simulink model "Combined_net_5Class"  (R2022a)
settings: Solver=FixedStepAuto  StartTime=0.0  StopTime=simtime  FixedStep=1  RelTol=1e-3
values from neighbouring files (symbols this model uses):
  simtime = length(SOC_CC{1, 1})    [Data_preparation.m]    (also in SimulationCycle.m = cell2mat(simtime_og(i)))
  SOH_predict = double(ans.SOHout(simtime))    [SimulationCycle.m]
undefined symbols (not defined in the file or in its folder): dSOC_mu_CC, dSOC_sig_CC, dv_mu_CC, dv_sig_CC, SOC_mu_CC, SOC_sig_CC, SOE_mu_CC, SOE_sig_CC
libraries: neural x183, deeplib x1
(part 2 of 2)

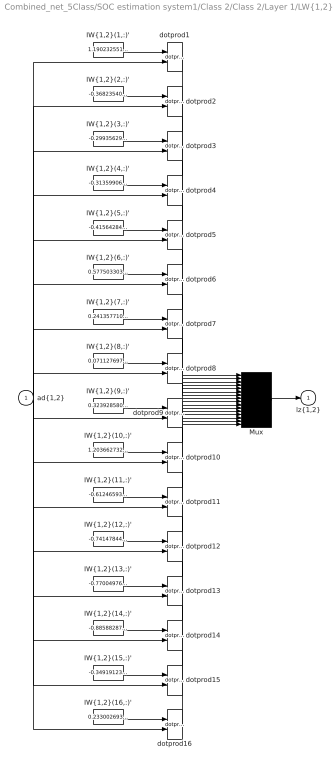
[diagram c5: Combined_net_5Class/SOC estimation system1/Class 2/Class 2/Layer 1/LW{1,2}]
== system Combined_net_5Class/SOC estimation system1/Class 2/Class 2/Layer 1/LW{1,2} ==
  "ad{1,2}" : Inport  PortDimensions=1  SampleTime=1
  "IW{1,2}(1,:)'" : Constant  Value=1.1902325515607079520208344547427259385585784912109375
  "IW{1,2}(10,:)'" : Constant  Value=1.2036627323236273046092037475318647921085357666015625
  "IW{1,2}(11,:)'" : Constant  Value=-0.61246593854063480222293947008438408374786376953125
  "IW{1,2}(12,:)'" : Constant  Value=-0.7414784419285955774370222570723854005336761474609375
  "IW{1,2}(13,:)'" : Constant  Value=-0.7700497660412211065050769320805557072162628173828125
  "IW{1,2}(14,:)'" : Constant  Value=-0.88588287817542854529762053061858750879764556884765625
  "IW{1,2}(15,:)'" : Constant  Value=-0.34919123068833413103817520095617510378360748291015625
  "IW{1,2}(16,:)'" : Constant  Value=0.23300269357094716138334433708223514258861541748046875
  "IW{1,2}(2,:)'" : Constant  Value=-0.368235400748596009012914009872474707663059234619140625
  "IW{1,2}(3,:)'" : Constant  Value=-0.299356293819304786207879942594445310533046722412109375
  "IW{1,2}(4,:)'" : Constant  Value=-0.313599061992354710692865182863897643983364105224609375
  "IW{1,2}(5,:)'" : Constant  Value=-0.415642846228695794774665728255058638751506805419921875
  "IW{1,2}(6,:)'" : Constant  Value=0.577503303425816572058693054714240133762359619140625
  "IW{1,2}(7,:)'" : Constant  Value=0.241357710985629025923770996087114326655864715576171875
  "IW{1,2}(8,:)'" : Constant  Value=0.07112769749609226810349582592607475817203521728515625
  "IW{1,2}(9,:)'" : Constant  Value=0.32392858033215443658292542750132270157337188720703125
  Mux : Mux  Inputs=16
  dotprod{1..16} (16 alike) : neural/Weight Functions/dotprod
  "lz{1,2}" : Outport
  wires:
  "IW{1,2}(1,:)'"/1 -> dotprod1/1
  "ad{1,2}"/1 -> dotprod1/2, dotprod2/2, dotprod3/2, dotprod4/2, dotprod5/2, dotprod6/2, dotprod7/2, dotprod8/2, dotprod9/2, dotprod10/2, dotprod11/2, dotprod12/2, dotprod13/2, dotprod14/2, dotprod15/2, dotprod16/2
  dotprod1/1 -> Mux/1
  "IW{1,2}(2,:)'"/1 -> dotprod2/1
  dotprod2/1 -> Mux/2
  "IW{1,2}(3,:)'"/1 -> dotprod3/1
  dotprod3/1 -> Mux/3
  "IW{1,2}(4,:)'"/1 -> dotprod4/1
  dotprod4/1 -> Mux/4
  "IW{1,2}(5,:)'"/1 -> dotprod5/1
  dotprod5/1 -> Mux/5
  "IW{1,2}(6,:)'"/1 -> dotprod6/1
  dotprod6/1 -> Mux/6
  "IW{1,2}(7,:)'"/1 -> dotprod7/1
  dotprod7/1 -> Mux/7
  "IW{1,2}(8,:)'"/1 -> dotprod8/1
  dotprod8/1 -> Mux/8
  "IW{1,2}(9,:)'"/1 -> dotprod9/1
  dotprod9/1 -> Mux/9
  "IW{1,2}(10,:)'"/1 -> dotprod10/1
  dotprod10/1 -> Mux/10
  "IW{1,2}(11,:)'"/1 -> dotprod11/1
  dotprod11/1 -> Mux/11
  "IW{1,2}(12,:)'"/1 -> dotprod12/1
  dotprod12/1 -> Mux/12
  "IW{1,2}(13,:)'"/1 -> dotprod13/1
  dotprod13/1 -> Mux/13
  "IW{1,2}(14,:)'"/1 -> dotprod14/1
  dotprod14/1 -> Mux/14
  "IW{1,2}(15,:)'"/1 -> dotprod15/1
  dotprod15/1 -> Mux/15
  "IW{1,2}(16,:)'"/1 -> dotprod16/1
  dotprod16/1 -> Mux/16
  Mux/1 -> "lz{1,2}"/1

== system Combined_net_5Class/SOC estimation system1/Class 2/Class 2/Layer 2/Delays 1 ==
  "p{2}" : Inport  PortDimensions=16  SampleTime=1
  mux : Mux  Inputs=1
  "pd{2,1}" : Outport
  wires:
  "p{2}"/1 -> mux/1
  mux/1 -> "pd{2,1}"/1

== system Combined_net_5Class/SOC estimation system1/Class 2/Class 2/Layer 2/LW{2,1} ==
  "ad{2,1}" : Inport  PortDimensions=16  SampleTime=1
  "IW{2,1}(1,:)'" : Constant  Value=[0.0007484560447357057992590068096205868641845881938934326171875;0.428302012501528384103011148908990435302257537841796875;-0.76136838015648000688173624439514242112636566162109375;-2.041090507574473189578156961943022906780242919921875;-1.5560079275295770617759671949897892773151397705078125;0.0002346400169689350358008528285580496230977587401866912841796875;0.00025834410646503381571437163444215912022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
  Mux : Mux  Inputs=1
  dotprod1 : neural/Weight Functions/dotprod
  "lz{2,1}" : Outport
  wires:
  "IW{2,1}(1,:)'"/1 -> dotprod1/1
  "ad{2,1}"/1 -> dotprod1/2
  dotprod1/1 -> Mux/1
  Mux/1 -> "lz{2,1}"/1

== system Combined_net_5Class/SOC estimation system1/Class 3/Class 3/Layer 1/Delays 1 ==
  "p{1}" : Inport  PortDimensions=3  SampleTime=1
  Delay 1 : UnitDelay  InitialCondition=pi_input_1_delayed_1
  mux : Mux  Inputs=2
  "pd{1,1}" : Outport
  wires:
  "p{1}"/1 -> Delay 1/1, mux/1
  Delay 1/1 -> mux/2
  mux/1 -> "pd{1,1}"/1

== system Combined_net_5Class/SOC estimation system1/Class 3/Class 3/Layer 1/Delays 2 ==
  "p{1}" : Inport  PortDimensions=1  SampleTime=1
  Delay 1 : UnitDelay  InitialCondition=ai_layer_2_delayed_1
  mux : Mux  Inputs=1
  "pd{1,2}" : Outport
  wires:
  "p{1}"/1 -> Delay 1/1
  Delay 1/1 -> mux/1
  mux/1 -> "pd{1,2}"/1

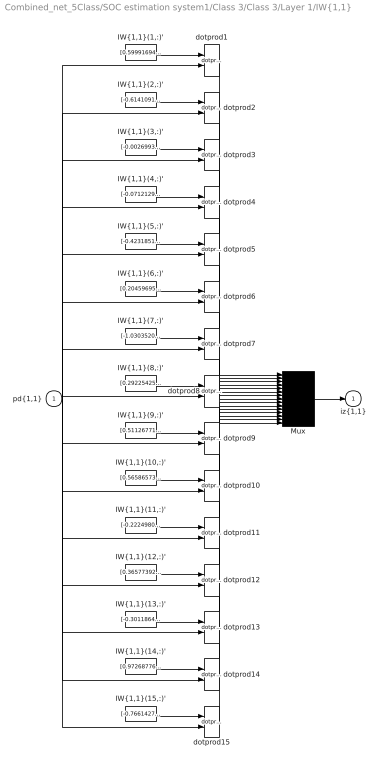
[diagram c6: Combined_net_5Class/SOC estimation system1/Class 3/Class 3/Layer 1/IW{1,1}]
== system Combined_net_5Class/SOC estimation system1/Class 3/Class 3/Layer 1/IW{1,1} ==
  "pd{1,1}" : Inport  PortDimensions=6  SampleTime=1
  "IW{1,1}(1,:)'" : Constant  Value=[0.5999169479734038912255300601827912032604217529296875;-0.380076540669565254848549784583155997097492218017578125;0.1751451252388635249079840150443487800657749176025390625;-0.581318210429382364878847511135973036289215087890625;0.388106402398013028420820091923815198242664337158203125;-0.1582639112277905157899482446737238205969333648681640625]
  "IW{1,1}(10,:)'" : Constant  Value=[0.565865737161032722468689826200716197490692138671875;-0.317511551991979945608335356155293993651866912841796875;0.71942713152451265301579041988588869571685791015625;-0.462730804023235353650278511850046925246715545654296875;-1.202674793055964475030350513407029211521148681640625;0.55537602898127691464225108575192280113697052001953125]
  "IW{1,1}(11,:)'" : Constant  Value=[-0.2224980177718796081620666882372461259365081787109375;0.0702328914913664392738468222887604497373104095458984375;-0.009460074424130826553636097742128185927867889404296875;0.2142790977150988707133905109003535471856594085693359375;-0.061660356138726273023120683092201943509280681610107421875;0.005611494475834051705309679647371012833900749683380126953125]
  "IW{1,1}(12,:)'" : Constant  Value=[0.3657739251182789974592424186994321644306182861328125;0.6914461290283744343554417355335317552089691162109375;0.004068878438489471026373589523927876143716275691986083984375;1.3485106085726688007753182318992912769317626953125;0.4634379678365778687521014944650232791900634765625;0.192226683034764700419572136524948291480541229248046875]
  "IW{1,1}(13,:)'" : Constant  Value=[-0.30118640813755892526870638903346844017505645751953125;0.460425695381792510207930035903700627386569976806640625;-0.07588917036400129323414631699051824398338794708251953125;1.275592741974297172902197416988201439380645751953125;-1.2831335957325811225615552757517434656620025634765625;-0.545358098592789719560869343695230782032012939453125]
  "IW{1,1}(14,:)'" : Constant  Value=[0.9726877674494531778037753610988147556781768798828125;0.95316906018628599905895271149347536265850067138671875;0.99977235084705673440197415402508340775966644287109375;1.0189879011847209344665543540031649172306060791015625;0.029875236411911858247503204211170668713748455047607421875;0.92824531588499337164677172040683217346668243408203125]
  "IW{1,1}(15,:)'" : Constant  Value=[-0.76614277146857745481867141279508359730243682861328125;0.790341085531665488161934263189323246479034423828125;1.167526088673049411426063670660369098186492919921875;0.52622667941697354176966427985462360084056854248046875;0.191965763204919703799333774441038258373737335205078125;-1.0897105784346734491663255539606325328350067138671875]
  "IW{1,1}(2,:)'" : Constant  Value=[-0.6141091996774454830898548607365228235721588134765625;-0.45684984466938971525706847387482412159442901611328125;0.9331109724455022291778050202992744743824005126953125;1.111277027417169716017042446765117347240447998046875;-0.27067200476342556658693183635477907955646514892578125;0.67860280468012346144490720689645968377590179443359375]
  "IW{1,1}(3,:)'" : Constant  Value=[-0.0026993480304873898080464389437338468269445002079010009765625;1.0531506048579901690942506320425309240818023681640625;-0.46427410659924195357461940147913992404937744140625;-0.06861728492135464596568539263898856006562709808349609375;-0.91250527596271047148235311397002078592777252197265625;0.44753207665025163120020579299307428300380706787109375]
  "IW{1,1}(4,:)'" : Constant  Value=[-0.0712129538313734100629659451442421413958072662353515625;-0.1639204208504933812928783254392328672111034393310546875;0.135310167368788591968353784977807663381099700927734375;0.07386291467043426539618167225853540003299713134765625;0.1754556862767355784882283842307515442371368408203125;-0.1304495041465366378385937196071608923375606536865234375]
  "IW{1,1}(5,:)'" : Constant  Value=[-0.42318514619345470872957548635895363986492156982421875;-0.14234031713342709668523866639588959515094757080078125;0.152692290242384565157607312357868067920207977294921875;0.418794176469951928698520760008250363171100616455078125;0.1525908291069372479942245490747154690325260162353515625;-0.1528109257425384337469864703962230123579502105712890625]
  "IW{1,1}(6,:)'" : Constant  Value=[0.2045969504738922584152760464348830282688140869140625;-0.1164344706358146630531535947739030234515666961669921875;0.0834505066323900368541188754534232430160045623779296875;-0.200411530848404739746371205910691060125827789306640625;0.1341741159839771324602253343982738442718982696533203125;-0.07641641521346569099204515396195347420871257781982421875]
  "IW{1,1}(7,:)'" : Constant  Value=[-1.030352081644546391459016376757062971591949462890625;-0.74553503133260579094354625340201891958713531494140625;-0.8059006155089887268871962078264914453029632568359375;-0.7160170072808520469465065616532228887081146240234375;-0.91338964557205015726282226751209236681461334228515625;0.644723544919552526977213346981443464756011962890625]
  "IW{1,1}(8,:)'" : Constant  Value=[0.29225425530896609327413671053363941609859466552734375;0.66285239858023015102617137017659842967987060546875;-0.7345223478168783071140524043585173785686492919921875;0.107853208325960736591042632426251657307147979736328125;-0.339523457818023122189998730391380377113819122314453125;0.96669615591649848962418900555348955094814300537109375]
  "IW{1,1}(9,:)'" : Constant  Value=[0.5112677113604837675353564918623305857181549072265625;0.133634811327623170829070886611589230597019195556640625;-0.15489111749693484920697983397985808551311492919921875;-0.506860225326407398682704297243617475032806396484375;-0.13691704481432598328183303237892687320709228515625;0.156147818778476887846551335314870811998844146728515625]
  Mux : Mux  Inputs=15
  dotprod{1..15} (15 alike) : neural/Weight Functions/dotprod
  "iz{1,1}" : Outport
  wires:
  "IW{1,1}(1,:)'"/1 -> dotprod1/1
  "pd{1,1}"/1 -> dotprod1/2, dotprod2/2, dotprod3/2, dotprod4/2, dotprod5/2, dotprod6/2, dotprod7/2, dotprod8/2, dotprod9/2, dotprod10/2, dotprod11/2, dotprod12/2, dotprod13/2, dotprod14/2, dotprod15/2
  dotprod1/1 -> Mux/1
  "IW{1,1}(2,:)'"/1 -> dotprod2/1
  dotprod2/1 -> Mux/2
  "IW{1,1}(3,:)'"/1 -> dotprod3/1
  dotprod3/1 -> Mux/3
  "IW{1,1}(4,:)'"/1 -> dotprod4/1
  dotprod4/1 -> Mux/4
  "IW{1,1}(5,:)'"/1 -> dotprod5/1
  dotprod5/1 -> Mux/5
  "IW{1,1}(6,:)'"/1 -> dotprod6/1
  dotprod6/1 -> Mux/6
  "IW{1,1}(7,:)'"/1 -> dotprod7/1
  dotprod7/1 -> Mux/7
  "IW{1,1}(8,:)'"/1 -> dotprod8/1
  dotprod8/1 -> Mux/8
  "IW{1,1}(9,:)'"/1 -> dotprod9/1
  dotprod9/1 -> Mux/9
  "IW{1,1}(10,:)'"/1 -> dotprod10/1
  dotprod10/1 -> Mux/10
  "IW{1,1}(11,:)'"/1 -> dotprod11/1
  dotprod11/1 -> Mux/11
  "IW{1,1}(12,:)'"/1 -> dotprod12/1
  dotprod12/1 -> Mux/12
  "IW{1,1}(13,:)'"/1 -> dotprod13/1
  dotprod13/1 -> Mux/13
  "IW{1,1}(14,:)'"/1 -> dotprod14/1
  dotprod14/1 -> Mux/14
  "IW{1,1}(15,:)'"/1 -> dotprod15/1
  dotprod15/1 -> Mux/15
  Mux/1 -> "iz{1,1}"/1

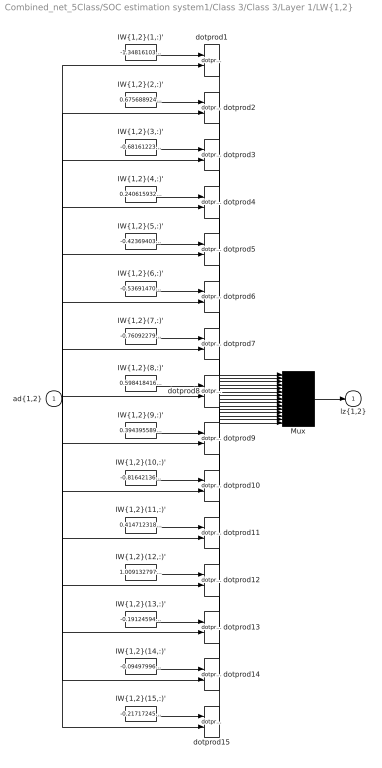
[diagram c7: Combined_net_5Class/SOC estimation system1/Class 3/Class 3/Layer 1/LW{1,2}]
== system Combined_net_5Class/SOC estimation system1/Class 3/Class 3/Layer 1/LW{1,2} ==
  "ad{1,2}" : Inport  PortDimensions=1  SampleTime=1
  "IW{1,2}(1,:)'" : Constant  Value=-1.3481610374089887383064478854066692292690277099609375
  "IW{1,2}(10,:)'" : Constant  Value=-0.81642136180247604215765022672712802886962890625
  "IW{1,2}(11,:)'" : Constant  Value=0.4147123184816428054233483635471202433109283447265625
  "IW{1,2}(12,:)'" : Constant  Value=1.0091327972796413359191092240507714450359344482421875
  "IW{1,2}(13,:)'" : Constant  Value=-0.1912459448195980293849771669556503184139728546142578125
  "IW{1,2}(14,:)'" : Constant  Value=-0.09497996596435183402906687888389569707214832305908203125
  "IW{1,2}(15,:)'" : Constant  Value=-0.217172454758892741200071441198815591633319854736328125
  "IW{1,2}(2,:)'" : Constant  Value=0.6756889243242161224856090484536252915859222412109375
  "IW{1,2}(3,:)'" : Constant  Value=-0.681612235710620684159266602364368736743927001953125
  "IW{1,2}(4,:)'" : Constant  Value=0.240615932200219706516008955077268183231353759765625
  "IW{1,2}(5,:)'" : Constant  Value=-0.42369403519754655906837115253438241779804229736328125
  "IW{1,2}(6,:)'" : Constant  Value=-0.53691470649667916159586411595228128135204315185546875
  "IW{1,2}(7,:)'" : Constant  Value=-0.76092279799986151100910092281992547214031219482421875
  "IW{1,2}(8,:)'" : Constant  Value=0.59841841694710395938017200023750774562358856201171875
  "IW{1,2}(9,:)'" : Constant  Value=0.394395589835405735446016706191585399210453033447265625
  Mux : Mux  Inputs=15
  dotprod{1..15} (15 alike) : neural/Weight Functions/dotprod
  "lz{1,2}" : Outport
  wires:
  "IW{1,2}(1,:)'"/1 -> dotprod1/1
  "ad{1,2}"/1 -> dotprod1/2, dotprod2/2, dotprod3/2, dotprod4/2, dotprod5/2, dotprod6/2, dotprod7/2, dotprod8/2, dotprod9/2, dotprod10/2, dotprod11/2, dotprod12/2, dotprod13/2, dotprod14/2, dotprod15/2
  dotprod1/1 -> Mux/1
  "IW{1,2}(2,:)'"/1 -> dotprod2/1
  dotprod2/1 -> Mux/2
  "IW{1,2}(3,:)'"/1 -> dotprod3/1
  dotprod3/1 -> Mux/3
  "IW{1,2}(4,:)'"/1 -> dotprod4/1
  dotprod4/1 -> Mux/4
  "IW{1,2}(5,:)'"/1 -> dotprod5/1
  dotprod5/1 -> Mux/5
  "IW{1,2}(6,:)'"/1 -> dotprod6/1
  dotprod6/1 -> Mux/6
  "IW{1,2}(7,:)'"/1 -> dotprod7/1
  dotprod7/1 -> Mux/7
  "IW{1,2}(8,:)'"/1 -> dotprod8/1
  dotprod8/1 -> Mux/8
  "IW{1,2}(9,:)'"/1 -> dotprod9/1
  dotprod9/1 -> Mux/9
  "IW{1,2}(10,:)'"/1 -> dotprod10/1
  dotprod10/1 -> Mux/10
  "IW{1,2}(11,:)'"/1 -> dotprod11/1
  dotprod11/1 -> Mux/11
  "IW{1,2}(12,:)'"/1 -> dotprod12/1
  dotprod12/1 -> Mux/12
  "IW{1,2}(13,:)'"/1 -> dotprod13/1
  dotprod13/1 -> Mux/13
  "IW{1,2}(14,:)'"/1 -> dotprod14/1
  dotprod14/1 -> Mux/14
  "IW{1,2}(15,:)'"/1 -> dotprod15/1
  dotprod15/1 -> Mux/15
  Mux/1 -> "lz{1,2}"/1

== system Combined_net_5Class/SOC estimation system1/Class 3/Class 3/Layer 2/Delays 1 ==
  "p{2}" : Inport  PortDimensions=15  SampleTime=1
  mux : Mux  Inputs=1
  "pd{2,1}" : Outport
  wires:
  "p{2}"/1 -> mux/1
  mux/1 -> "pd{2,1}"/1

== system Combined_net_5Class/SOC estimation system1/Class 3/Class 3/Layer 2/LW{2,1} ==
  "ad{2,1}" : Inport  PortDimensions=15  SampleTime=1
  "IW{2,1}(1,:)'" : Constant  Value=[-0.08703702797859691475679255745490081608295440673828125;-2.752635990016915270455800934801260382300824858248233795166015625e-05;-0.06954371822944267755861602609002147801220417022705078125;1.0956141479609495803515528677962720394134521484375;-0.55686157695599802774921727177570573985576629638671875;-0.58502372249182155172775310347788035869598388671875;-0.000143661824552710105798794537612650401570135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
  Mux : Mux  Inputs=1
  dotprod1 : neural/Weight Functions/dotprod
  "lz{2,1}" : Outport
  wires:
  "IW{2,1}(1,:)'"/1 -> dotprod1/1
  "ad{2,1}"/1 -> dotprod1/2
  dotprod1/1 -> Mux/1
  Mux/1 -> "lz{2,1}"/1

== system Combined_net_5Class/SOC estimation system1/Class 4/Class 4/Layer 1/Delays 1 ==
  "p{1}" : Inport  PortDimensions=3  SampleTime=1
  Delay 1 : UnitDelay  InitialCondition=pi_input_1_delayed_1
  mux : Mux  Inputs=2
  "pd{1,1}" : Outport
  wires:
  "p{1}"/1 -> Delay 1/1, mux/1
  Delay 1/1 -> mux/2
  mux/1 -> "pd{1,1}"/1

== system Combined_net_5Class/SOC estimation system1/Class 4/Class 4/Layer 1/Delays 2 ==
  "p{1}" : Inport  PortDimensions=1  SampleTime=1
  Delay 1 : UnitDelay  InitialCondition=ai_layer_2_delayed_1
  mux : Mux  Inputs=1
  "pd{1,2}" : Outport
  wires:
  "p{1}"/1 -> Delay 1/1
  Delay 1/1 -> mux/1
  mux/1 -> "pd{1,2}"/1

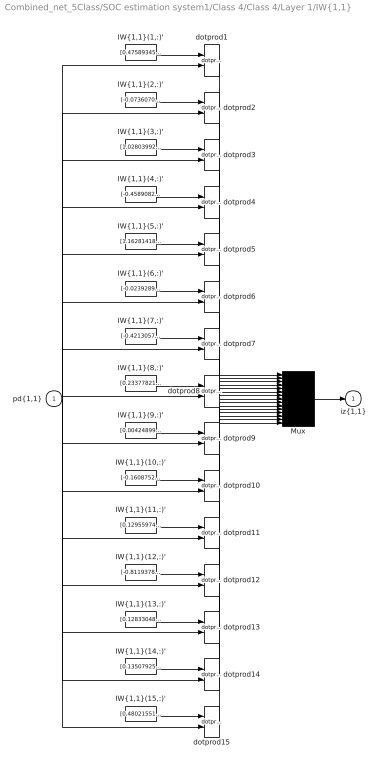
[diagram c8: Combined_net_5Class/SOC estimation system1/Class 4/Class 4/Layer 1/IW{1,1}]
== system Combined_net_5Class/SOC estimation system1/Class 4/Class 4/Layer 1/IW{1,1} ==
  "pd{1,1}" : Inport  PortDimensions=6  SampleTime=1
  "IW{1,1}(1,:)'" : Constant  Value=[0.47589345629772805690294035230181179940700531005859375;-0.0925483739468922206317103018591296859085559844970703125;0.2214082445588193837071600000854232348501682281494140625;-0.55827092134025979586198218385106883943080902099609375;0.371810857100516034545734100902336649596691131591796875;-0.2254368218410331137224744679770083166658878326416015625]
  "IW{1,1}(10,:)'" : Constant  Value=[-0.160875254906906739460481503556366078555583953857421875;1.25545079189343056214056559838354587554931640625;0.82227860729125878958001294449786655604839324951171875;0.68907741180449144646757986265583895146846771240234375;0.4760328509045412825884113772190175950527191162109375;0.56508116495892657393795843745465390384197235107421875]
  "IW{1,1}(11,:)'" : Constant  Value=[0.1295597493069054195746758750829030759632587432861328125;-0.7027206554819176442805428450810723006725311279296875;0.01048723608229113792023046158874421962536871433258056640625;-0.12144154837862077001009453169899643398821353912353515625;0.6716008198873224532832182376296259462833404541015625;-0.01110885898004046294651470105918633635155856609344482421875]
  "IW{1,1}(12,:)'" : Constant  Value=[-0.81193787871365652453192751636379398405551910400390625;0.052979932259121904902787747460024547763168811798095703125;-0.85219833133312661299640922152320854365825653076171875;-1.2892547171023380769838695414364337921142578125;0.2888823598052636665300951790413819253444671630859375;0.95946581169378186704221889158361591398715972900390625]
  "IW{1,1}(13,:)'" : Constant  Value=[0.1283304883345246227843716724237310700118541717529296875;-1.0510763220670835682568622360122390091419219970703125;-0.00978941947522312012897049982029784587211906909942626953125;-0.105105436360953097274517631376511417329311370849609375;0.97365481852998014833389106570393778383731842041015625;0.0094649789740008476168764417479906114749610424041748046875]
  "IW{1,1}(14,:)'" : Constant  Value=[0.13507925712913604332499062365968711674213409423828125;1.3465969135515039045714047460933215916156768798828125;0.037650426815895358945152082696949946694076061248779296875;-0.24636647845154213687379751718253828585147857666015625;-1.098457241066270295704043746809475123882293701171875;-0.031137150955768626292563538981994497589766979217529296875]
  "IW{1,1}(15,:)'" : Constant  Value=[0.4802155133064338610182630873168818652629852294921875;1.0470200768443069794244593140319921076297760009765625;0.91055601721542556159505465984693728387355804443359375;-0.66866377880541183476026390053448267281055450439453125;-0.75655368821547364088786480351700447499752044677734375;-0.95651666815045055525246198158129118382930755615234375]
  "IW{1,1}(2,:)'" : Constant  Value=[-0.0736070813836286197417990706526325084269046783447265625;-0.67197103462730478629083563646418042480945587158203125;-0.00236642124665641107039704138514935038983821868896484375;0.07921471418529670016628330131425173021852970123291015625;0.6545789596461053516662786933011375367641448974609375;0.0020292910834603093174488552818957032286562025547027587890625]
  "IW{1,1}(3,:)'" : Constant  Value=[1.0280399260244188486268512860988266766071319580078125;-0.27942027557096482670573323048301972448825836181640625;-0.0892909183637599357385994380820193327963352203369140625;-0.453795175317589005725693596104974858462810516357421875;-0.576024269824537693551746997400186955928802490234375;0.0560093918069750340560375434506568126380443572998046875]
  "IW{1,1}(4,:)'" : Constant  Value=[-0.45890827140267054229383347774273715913295745849609375;-0.10751401854145288539132963023803313262760639190673828125;-0.64165865824107537473963702723267488181591033935546875;-0.340283065341602519726649234144133515655994415283203125;-0.98025402834946107066826925802160985767841339111328125;0.62624537413127134843904286753968335688114166259765625]
  "IW{1,1}(5,:)'" : Constant  Value=[1.1628141888303853423991540694260038435459136962890625;0.83995134932578408015757531757117249071598052978515625;-0.74679131201013160268331603219849057495594024658203125;0.9695999053100703424235007332754321396350860595703125;0.81385399734751906475338500968064181506633758544921875;-0.3506986361075525859831714114989154040813446044921875]
  "IW{1,1}(6,:)'" : Constant  Value=[-0.0239289753768265299471718066115499823354184627532958984375;-0.1904667274971808821337759809466660954058170318603515625;-0.000510908803777701645172648614590116267208941280841827392578125;0.0240816257388850353537979032125804224051535129547119140625;0.1879091054420398976265715873523731715977191925048828125;0.0004578940268036963377740189429232486872933804988861083984375]
  "IW{1,1}(7,:)'" : Constant  Value=[-0.421305718572614562589251363533549010753631591796875;-1.638905485601443334786608829745091497898101806640625;-0.060187823819410381231964635162512422539293766021728515625;-1.17351884861722055575228296220302581787109375;-0.5845835467423563525102281346335075795650482177734375;-0.3167451786432484706068635205156169831752777099609375]
  "IW{1,1}(8,:)'" : Constant  Value=[0.2337782179630895351696295847432338632643222808837890625;0.7693182498319444118095589146832935512065887451171875;-0.98242689204637134725572877869126386940479278564453125;0.8006839507068070904693968259380199015140533447265625;0.98439935115788335107112061450607143342494964599609375;-0.69129174189053410604088867330574430525302886962890625]
  "IW{1,1}(9,:)'" : Constant  Value=[0.004248991871379369407446535689132360857911407947540283203125;-0.0532891868962488413075107018812559545040130615234375;0.000351429482347537128043846177405384878511540591716766357421875;-0.0028150212982930044626483923053683611215092241764068603515625;0.049523321139780758504134183795031276531517505645751953125;-0.00042134089612695592615143613812733747181482613086700439453125]
  Mux : Mux  Inputs=15
  dotprod{1..15} (15 alike) : neural/Weight Functions/dotprod
  "iz{1,1}" : Outport
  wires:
  "IW{1,1}(1,:)'"/1 -> dotprod1/1
  "pd{1,1}"/1 -> dotprod1/2, dotprod2/2, dotprod3/2, dotprod4/2, dotprod5/2, dotprod6/2, dotprod7/2, dotprod8/2, dotprod9/2, dotprod10/2, dotprod11/2, dotprod12/2, dotprod13/2, dotprod14/2, dotprod15/2
  dotprod1/1 -> Mux/1
  "IW{1,1}(2,:)'"/1 -> dotprod2/1
  dotprod2/1 -> Mux/2
  "IW{1,1}(3,:)'"/1 -> dotprod3/1
  dotprod3/1 -> Mux/3
  "IW{1,1}(4,:)'"/1 -> dotprod4/1
  dotprod4/1 -> Mux/4
  "IW{1,1}(5,:)'"/1 -> dotprod5/1
  dotprod5/1 -> Mux/5
  "IW{1,1}(6,:)'"/1 -> dotprod6/1
  dotprod6/1 -> Mux/6
  "IW{1,1}(7,:)'"/1 -> dotprod7/1
  dotprod7/1 -> Mux/7
  "IW{1,1}(8,:)'"/1 -> dotprod8/1
  dotprod8/1 -> Mux/8
  "IW{1,1}(9,:)'"/1 -> dotprod9/1
  dotprod9/1 -> Mux/9
  "IW{1,1}(10,:)'"/1 -> dotprod10/1
  dotprod10/1 -> Mux/10
  "IW{1,1}(11,:)'"/1 -> dotprod11/1
  dotprod11/1 -> Mux/11
  "IW{1,1}(12,:)'"/1 -> dotprod12/1
  dotprod12/1 -> Mux/12
  "IW{1,1}(13,:)'"/1 -> dotprod13/1
  dotprod13/1 -> Mux/13
  "IW{1,1}(14,:)'"/1 -> dotprod14/1
  dotprod14/1 -> Mux/14
  "IW{1,1}(15,:)'"/1 -> dotprod15/1
  dotprod15/1 -> Mux/15
  Mux/1 -> "iz{1,1}"/1

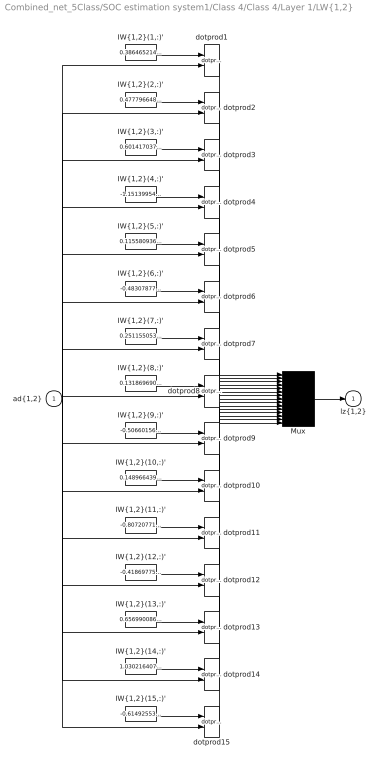
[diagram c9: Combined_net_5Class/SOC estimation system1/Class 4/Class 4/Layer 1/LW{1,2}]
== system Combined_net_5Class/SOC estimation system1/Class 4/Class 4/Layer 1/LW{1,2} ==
  "ad{1,2}" : Inport  PortDimensions=1  SampleTime=1
  "IW{1,2}(1,:)'" : Constant  Value=0.386465214186513750238560760408290661871433258056640625
  "IW{1,2}(10,:)'" : Constant  Value=0.1489664399058193977598563151332200504839420318603515625
  "IW{1,2}(11,:)'" : Constant  Value=-0.80720771417523540236516055301763117313385009765625
  "IW{1,2}(12,:)'" : Constant  Value=-0.418697757909935630582509702435345388948917388916015625
  "IW{1,2}(13,:)'" : Constant  Value=0.65699008647876844246837890750612132251262664794921875
  "IW{1,2}(14,:)'" : Constant  Value=1.0302164070648329730062187081784941256046295166015625
  "IW{1,2}(15,:)'" : Constant  Value=-0.6149255364488237507458734398824162781238555908203125
  "IW{1,2}(2,:)'" : Constant  Value=0.4777966485166749155411025640205480158329010009765625
  "IW{1,2}(3,:)'" : Constant  Value=0.60141703706550331265390241242130286991596221923828125
  "IW{1,2}(4,:)'" : Constant  Value=-1.151399547135881551440661496599204838275909423828125
  "IW{1,2}(5,:)'" : Constant  Value=0.11558093686261845800533620831629377789795398712158203125
  "IW{1,2}(6,:)'" : Constant  Value=-0.483078779207699204878423415721044875681400299072265625
  "IW{1,2}(7,:)'" : Constant  Value=0.251155053057356136836375526399933733046054840087890625
  "IW{1,2}(8,:)'" : Constant  Value=0.131869690192287725150066535206860862672328948974609375
  "IW{1,2}(9,:)'" : Constant  Value=-0.50660156135882938865933056149515323340892791748046875
  Mux : Mux  Inputs=15
  dotprod{1..15} (15 alike) : neural/Weight Functions/dotprod
  "lz{1,2}" : Outport
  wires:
  "IW{1,2}(1,:)'"/1 -> dotprod1/1
  "ad{1,2}"/1 -> dotprod1/2, dotprod2/2, dotprod3/2, dotprod4/2, dotprod5/2, dotprod6/2, dotprod7/2, dotprod8/2, dotprod9/2, dotprod10/2, dotprod11/2, dotprod12/2, dotprod13/2, dotprod14/2, dotprod15/2
  dotprod1/1 -> Mux/1
  "IW{1,2}(2,:)'"/1 -> dotprod2/1
  dotprod2/1 -> Mux/2
  "IW{1,2}(3,:)'"/1 -> dotprod3/1
  dotprod3/1 -> Mux/3
  "IW{1,2}(4,:)'"/1 -> dotprod4/1
  dotprod4/1 -> Mux/4
  "IW{1,2}(5,:)'"/1 -> dotprod5/1
  dotprod5/1 -> Mux/5
  "IW{1,2}(6,:)'"/1 -> dotprod6/1
  dotprod6/1 -> Mux/6
  "IW{1,2}(7,:)'"/1 -> dotprod7/1
  dotprod7/1 -> Mux/7
  "IW{1,2}(8,:)'"/1 -> dotprod8/1
  dotprod8/1 -> Mux/8
  "IW{1,2}(9,:)'"/1 -> dotprod9/1
  dotprod9/1 -> Mux/9
  "IW{1,2}(10,:)'"/1 -> dotprod10/1
  dotprod10/1 -> Mux/10
  "IW{1,2}(11,:)'"/1 -> dotprod11/1
  dotprod11/1 -> Mux/11
  "IW{1,2}(12,:)'"/1 -> dotprod12/1
  dotprod12/1 -> Mux/12
  "IW{1,2}(13,:)'"/1 -> dotprod13/1
  dotprod13/1 -> Mux/13
  "IW{1,2}(14,:)'"/1 -> dotprod14/1
  dotprod14/1 -> Mux/14
  "IW{1,2}(15,:)'"/1 -> dotprod15/1
  dotprod15/1 -> Mux/15
  Mux/1 -> "lz{1,2}"/1

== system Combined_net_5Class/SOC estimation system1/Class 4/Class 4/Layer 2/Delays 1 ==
  "p{2}" : Inport  PortDimensions=15  SampleTime=1
  mux : Mux  Inputs=1
  "pd{2,1}" : Outport
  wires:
  "p{2}"/1 -> mux/1
  mux/1 -> "pd{2,1}"/1

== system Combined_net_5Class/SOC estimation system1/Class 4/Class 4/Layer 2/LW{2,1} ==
  "ad{2,1}" : Inport  PortDimensions=15  SampleTime=1
  "IW{2,1}(1,:)'" : Constant  Value=[0.277055266825274149056212991126812994480133056640625;0.371118023797417151410371616293559782207012176513671875;0.0115574154567635416224202771218187990598380565643310546875;-0.0001853056881339489405692566581507207956747151911258697509765625;-1.14632749146578577289644525205591918393110972829163074493408203125e-06;-1.1361132075220792270187075700960122048854827880859375;3.4575884736824709516332665426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
  Mux : Mux  Inputs=1
  dotprod1 : neural/Weight Functions/dotprod
  "lz{2,1}" : Outport
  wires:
  "IW{2,1}(1,:)'"/1 -> dotprod1/1
  "ad{2,1}"/1 -> dotprod1/2
  dotprod1/1 -> Mux/1
  Mux/1 -> "lz{2,1}"/1

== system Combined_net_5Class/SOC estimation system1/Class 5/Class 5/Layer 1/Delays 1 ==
  "p{1}" : Inport  PortDimensions=3  SampleTime=1
  Delay 1 : UnitDelay  InitialCondition=pi_input_1_delayed_1
  mux : Mux  Inputs=2
  "pd{1,1}" : Outport
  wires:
  "p{1}"/1 -> Delay 1/1, mux/1
  Delay 1/1 -> mux/2
  mux/1 -> "pd{1,1}"/1

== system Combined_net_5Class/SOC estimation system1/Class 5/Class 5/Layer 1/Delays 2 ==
  "p{1}" : Inport  PortDimensions=1  SampleTime=1
  Delay 1 : UnitDelay  InitialCondition=ai_layer_2_delayed_1
  mux : Mux  Inputs=1
  "pd{1,2}" : Outport
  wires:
  "p{1}"/1 -> Delay 1/1
  Delay 1/1 -> mux/1
  mux/1 -> "pd{1,2}"/1

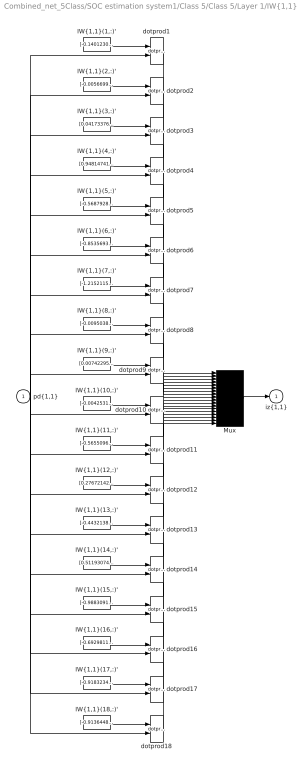
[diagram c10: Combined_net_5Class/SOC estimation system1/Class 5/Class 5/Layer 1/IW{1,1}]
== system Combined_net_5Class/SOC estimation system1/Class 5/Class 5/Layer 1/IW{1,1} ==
  "pd{1,1}" : Inport  PortDimensions=6  SampleTime=1
  "IW{1,1}(1,:)'" : Constant  Value=[-0.1401230434751131459503170617608702741563320159912109375;0.09804398778615174003814303205217584036290645599365234375;-0.650864888767997751273242101888172328472137451171875;-0.049125248265707625872078523343589040450751781463623046875;0.493880659636385888067167115877964533865451812744140625;0.5318910777836773906557255031657405197620391845703125]
  "IW{1,1}(10,:)'" : Constant  Value=[-0.004253125137399535286852891857733993674628436565399169921875;0.29351396381755401332469546105130575597286224365234375;0.41740709390548824675448713605874218046665191650390625;0.09159101661829448237650552755440003238618373870849609375;-0.60156066265264140913160417767358012497425079345703125;-0.351859991912801761682061396641074679791927337646484375]
  "IW{1,1}(11,:)'" : Constant  Value=[-0.5655096500572920348304251092486083507537841796875;-1.03581042296727243723353240056894719600677490234375;-0.0414856024920069177408521454708534292876720428466796875;-1.5427709526310680043792444848804734647274017333984375;0.8523229396129992085917592703481204807758331298828125;-0.61026511014981077440921808374696411192417144775390625]
  "IW{1,1}(12,:)'" : Constant  Value=[0.276721426407887050036293885568738915026187896728515625;1.3349675233139119967518126941286027431488037109375;-0.0705178521016570913904075723621645011007785797119140625;-0.85394119414376901122665231014252640306949615478515625;0.1634447175296280807543780611013062298297882080078125;0.263866012049225273639052602447918616235256195068359375]
  "IW{1,1}(13,:)'" : Constant  Value=[-0.443213825982611331344429572709486819803714752197265625;0.07417879621131158451863285563376848585903644561767578125;0.091985121041477102554750899798818863928318023681640625;-0.9292473782737735721326544080511666834354400634765625;0.0273930683487181268753740681631825282238423824310302734375;-0.350421183561417770579993202773039229214191436767578125]
  "IW{1,1}(14,:)'" : Constant  Value=[0.51193074350790779281084041940630413591861724853515625;0.461426155934119230916934384367777965962886810302734375;0.2933423174624507634433712155441753566265106201171875;-0.999552528081245394986353858257643878459930419921875;-0.6171983935838787349581480157212354242801666259765625;-0.72218597194273692618793347719474695622920989990234375]
  "IW{1,1}(15,:)'" : Constant  Value=[-0.98830910004782468458728317273198626935482025146484375;-0.59206284926831909132260989281348884105682373046875;-0.1507131259827427793851484238984994590282440185546875;0.790631607545934311787050319253467023372650146484375;-1.055723688879461885647970120771788060665130615234375;-0.0813493562885934939910015373243368230760097503662109375]
  "IW{1,1}(16,:)'" : Constant  Value=[-0.69298110213156582926075088835204951465129852294921875;-0.55617690153965415600367805382120423018932342529296875;0.789902499847435546342921952600590884685516357421875;-0.98445106997453424302335633910843171179294586181640625;-0.2168932212369263645701522591480170376598834991455078125;-0.389833407553313138205197674324153922498226165771484375]
  "IW{1,1}(17,:)'" : Constant  Value=[-0.9183234277123932809416828604298643767833709716796875;-0.7411934283578387461233205613098107278347015380859375;-0.07261949038330185735024002724458114244043827056884765625;1.262877414926813823825568761094473302364349365234375;-0.48332864838868949686201403892482630908489227294921875;0.493187056811075219542317427112720906734466552734375]
  "IW{1,1}(18,:)'" : Constant  Value=[-0.9136448473848506335315278192865662276744842529296875;-0.83803867452566171980521403384045697748661041259765625;-0.06286424511210954302331543885884457267820835113525390625;1.2622621532108173614261659167823381721973419189453125;-0.39783817259554865586324012838304042816162109375;0.485497996657707375778301184254814870655536651611328125]
  "IW{1,1}(2,:)'" : Constant  Value=[-0.00566995694964670012006013877225996111519634723663330078125;-0.05511895904537218726648717392890830524265766143798828125;-0.23953368882451153698553980575525201857089996337890625;-0.048183206110769781493896601887172437272965908050537109375;0.239840751795701578874542292396654374897480010986328125;0.2009326012946475170650728614418767392635345458984375]
  "IW{1,1}(3,:)'" : Constant  Value=[0.04173376720858455735108094586394145153462886810302734375;0.374299495454836428365297251730225980281829833984375;0.1816860582433664494939051792243844829499721527099609375;0.0241588600291725193180969455397644196636974811553955078125;-0.58044387247013862207722922903485596179962158203125;-0.148136032249187532539025369260343722999095916748046875]
  "IW{1,1}(4,:)'" : Constant  Value=[0.94814741138349922788819412744487635791301727294921875;-0.47915002049430144293040712000220082700252532958984375;0.66988762246262345545488869902328588068485260009765625;0.2465776080757873522930623266802285797894001007080078125;0.45954570011964313014374283739016391336917877197265625;-0.025936623130433246464665586472619906999170780181884765625]
  "IW{1,1}(5,:)'" : Constant  Value=[-0.56879283836661631568176744622178375720977783203125;-0.56665032129272685512688667586189694702625274658203125;0.5017524731900431245179561301483772695064544677734375;-0.6757125982821901022390420621377415955066680908203125;0.403757277203605269288999579657684080302715301513671875;1.394891767333193310918204588233493268489837646484375]
  "IW{1,1}(6,:)'" : Constant  Value=[-0.8535693304909879319808396758162416517734527587890625;-0.1445803727679269012895701962406747043132781982421875;0.94962006493938699858148311250261031091213226318359375;-0.6958758564855933581583258273894898593425750732421875;0.69299647350054083272397065229597501456737518310546875;-0.4961428253686761546958905455539934337139129638671875]
  "IW{1,1}(7,:)'" : Constant  Value=[-1.215211566484807992338801341247744858264923095703125;-0.50710572162662492790019541644142009317874908447265625;0.53910417232163643230791194582707248628139495849609375;-1.3870074518725916679073861814686097204685211181640625;0.004168099557994189678644669783125209505669772624969482421875;-0.70547927472520688407797706531709991395473480224609375]
  "IW{1,1}(8,:)'" : Constant  Value=[-0.00950381828604053048581423723817351856268942356109619140625;0.056971293158991943850200101451264345087110996246337890625;-0.097583977334529337088753209172864444553852081298828125;-0.0128046313446012784142968854439459391869604587554931640625;0.0155016043180136627033238738704312709160149097442626953125;0.0804500636322046103199312483411631546914577484130859375]
  "IW{1,1}(9,:)'" : Constant  Value=[0.00742295551394898424357737809486934565939009189605712890625;-0.046797500999922685138709965713132987730205059051513671875;0.074769816342900530248272161770728416740894317626953125;0.00921788818793813947982673795422670082189142704010009765625;-0.00852458168770966161209567957257604575715959072113037109375;-0.061701940636885312108095291705467388965189456939697265625]
  Mux : Mux  Inputs=18
  dotprod{1..18} (18 alike) : neural/Weight Functions/dotprod
  "iz{1,1}" : Outport
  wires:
  "IW{1,1}(1,:)'"/1 -> dotprod1/1
  "pd{1,1}"/1 -> dotprod1/2, dotprod2/2, dotprod3/2, dotprod4/2, dotprod5/2, dotprod6/2, dotprod7/2, dotprod8/2, dotprod9/2, dotprod10/2, dotprod11/2, dotprod12/2, dotprod13/2, dotprod14/2, dotprod15/2, dotprod16/2, dotprod17/2, dotprod18/2
  dotprod1/1 -> Mux/1
  "IW{1,1}(2,:)'"/1 -> dotprod2/1
  dotprod2/1 -> Mux/2
  "IW{1,1}(3,:)'"/1 -> dotprod3/1
  dotprod3/1 -> Mux/3
  "IW{1,1}(4,:)'"/1 -> dotprod4/1
  dotprod4/1 -> Mux/4
  "IW{1,1}(5,:)'"/1 -> dotprod5/1
  dotprod5/1 -> Mux/5
  "IW{1,1}(6,:)'"/1 -> dotprod6/1
  dotprod6/1 -> Mux/6
  "IW{1,1}(7,:)'"/1 -> dotprod7/1
  dotprod7/1 -> Mux/7
  "IW{1,1}(8,:)'"/1 -> dotprod8/1
  dotprod8/1 -> Mux/8
  "IW{1,1}(9,:)'"/1 -> dotprod9/1
  dotprod9/1 -> Mux/9
  "IW{1,1}(10,:)'"/1 -> dotprod10/1
  dotprod10/1 -> Mux/10
  "IW{1,1}(11,:)'"/1 -> dotprod11/1
  dotprod11/1 -> Mux/11
  "IW{1,1}(12,:)'"/1 -> dotprod12/1
  dotprod12/1 -> Mux/12
  "IW{1,1}(13,:)'"/1 -> dotprod13/1
  dotprod13/1 -> Mux/13
  "IW{1,1}(14,:)'"/1 -> dotprod14/1
  dotprod14/1 -> Mux/14
  "IW{1,1}(15,:)'"/1 -> dotprod15/1
  dotprod15/1 -> Mux/15
  "IW{1,1}(16,:)'"/1 -> dotprod16/1
  dotprod16/1 -> Mux/16
  "IW{1,1}(17,:)'"/1 -> dotprod17/1
  dotprod17/1 -> Mux/17
  "IW{1,1}(18,:)'"/1 -> dotprod18/1
  dotprod18/1 -> Mux/18
  Mux/1 -> "iz{1,1}"/1

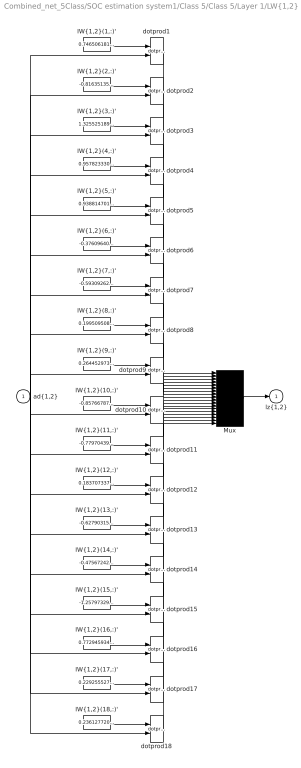
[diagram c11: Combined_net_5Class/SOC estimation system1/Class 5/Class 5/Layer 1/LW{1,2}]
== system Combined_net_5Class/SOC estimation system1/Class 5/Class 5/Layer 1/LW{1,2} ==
  "ad{1,2}" : Inport  PortDimensions=1  SampleTime=1
  "IW{1,2}(1,:)'" : Constant  Value=0.74650618165794302427684669964946806430816650390625
  "IW{1,2}(10,:)'" : Constant  Value=-0.857667873992931983906373716308735311031341552734375
  "IW{1,2}(11,:)'" : Constant  Value=-0.77970439722816553551609786154585890471935272216796875
  "IW{1,2}(12,:)'" : Constant  Value=0.183707337369911238855735291508608497679233551025390625
  "IW{1,2}(13,:)'" : Constant  Value=-0.62790315350138092842513515279279090464115142822265625
  "IW{1,2}(14,:)'" : Constant  Value=-0.4756724216767820312412595740170218050479888916015625
  "IW{1,2}(15,:)'" : Constant  Value=-1.2579732939525725132767774994135834276676177978515625
  "IW{1,2}(16,:)'" : Constant  Value=0.77294593488091900557179769748472608625888824462890625
  "IW{1,2}(17,:)'" : Constant  Value=0.229255527918000356901728764569270424544811248779296875
  "IW{1,2}(18,:)'" : Constant  Value=0.236127720819241992966652787799830548465251922607421875
  "IW{1,2}(2,:)'" : Constant  Value=-0.816351351809472713938475862960331141948699951171875
  "IW{1,2}(3,:)'" : Constant  Value=1.3255251899563422757211128555354662239551544189453125
  "IW{1,2}(4,:)'" : Constant  Value=0.957823330549129270394814739120192825794219970703125
  "IW{1,2}(5,:)'" : Constant  Value=0.938814701924564953827712088241241872310638427734375
  "IW{1,2}(6,:)'" : Constant  Value=-0.376096402206848645644043926949962042272090911865234375
  "IW{1,2}(7,:)'" : Constant  Value=-0.59309262343324908872688183691934682428836822509765625
  "IW{1,2}(8,:)'" : Constant  Value=0.1995095083869170837775897098254063166677951812744140625
  "IW{1,2}(9,:)'" : Constant  Value=0.2644529731292568630607320301351137459278106689453125
  Mux : Mux  Inputs=18
  dotprod{1..18} (18 alike) : neural/Weight Functions/dotprod
  "lz{1,2}" : Outport
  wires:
  "IW{1,2}(1,:)'"/1 -> dotprod1/1
  "ad{1,2}"/1 -> dotprod1/2, dotprod2/2, dotprod3/2, dotprod4/2, dotprod5/2, dotprod6/2, dotprod7/2, dotprod8/2, dotprod9/2, dotprod10/2, dotprod11/2, dotprod12/2, dotprod13/2, dotprod14/2, dotprod15/2, dotprod16/2, dotprod17/2, dotprod18/2
  dotprod1/1 -> Mux/1
  "IW{1,2}(2,:)'"/1 -> dotprod2/1
  dotprod2/1 -> Mux/2
  "IW{1,2}(3,:)'"/1 -> dotprod3/1
  dotprod3/1 -> Mux/3
  "IW{1,2}(4,:)'"/1 -> dotprod4/1
  dotprod4/1 -> Mux/4
  "IW{1,2}(5,:)'"/1 -> dotprod5/1
  dotprod5/1 -> Mux/5
  "IW{1,2}(6,:)'"/1 -> dotprod6/1
  dotprod6/1 -> Mux/6
  "IW{1,2}(7,:)'"/1 -> dotprod7/1
  dotprod7/1 -> Mux/7
  "IW{1,2}(8,:)'"/1 -> dotprod8/1
  dotprod8/1 -> Mux/8
  "IW{1,2}(9,:)'"/1 -> dotprod9/1
  dotprod9/1 -> Mux/9
  "IW{1,2}(10,:)'"/1 -> dotprod10/1
  dotprod10/1 -> Mux/10
  "IW{1,2}(11,:)'"/1 -> dotprod11/1
  dotprod11/1 -> Mux/11
  "IW{1,2}(12,:)'"/1 -> dotprod12/1
  dotprod12/1 -> Mux/12
  "IW{1,2}(13,:)'"/1 -> dotprod13/1
  dotprod13/1 -> Mux/13
  "IW{1,2}(14,:)'"/1 -> dotprod14/1
  dotprod14/1 -> Mux/14
  "IW{1,2}(15,:)'"/1 -> dotprod15/1
  dotprod15/1 -> Mux/15
  "IW{1,2}(16,:)'"/1 -> dotprod16/1
  dotprod16/1 -> Mux/16
  "IW{1,2}(17,:)'"/1 -> dotprod17/1
  dotprod17/1 -> Mux/17
  "IW{1,2}(18,:)'"/1 -> dotprod18/1
  dotprod18/1 -> Mux/18
  Mux/1 -> "lz{1,2}"/1

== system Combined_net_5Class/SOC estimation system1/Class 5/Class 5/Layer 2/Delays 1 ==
  "p{2}" : Inport  PortDimensions=18  SampleTime=1
  mux : Mux  Inputs=1
  "pd{2,1}" : Outport
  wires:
  "p{2}"/1 -> mux/1
  mux/1 -> "pd{2,1}"/1

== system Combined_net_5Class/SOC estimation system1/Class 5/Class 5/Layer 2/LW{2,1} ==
  "ad{2,1}" : Inport  PortDimensions=18  SampleTime=1
  "IW{2,1}(1,:)'" : Constant  Value=[0.0278759648941551800571669872397251310758292675018310546875;-0.1807291869353111757323659958274220116436481475830078125;0.044520908843115540587387357618354144506156444549560546875;0.00020185454198865700734845385344584656195365823805332183837890625;2.398147982544406617115562152520169547642581164836883544921875e-05;-0.000506729432523865823585762502290208431077189743518829345703125;0.000183181848600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
  Mux : Mux  Inputs=1
  dotprod1 : neural/Weight Functions/dotprod
  "lz{2,1}" : Outport
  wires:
  "IW{2,1}(1,:)'"/1 -> dotprod1/1
  "ad{2,1}"/1 -> dotprod1/2
  dotprod1/1 -> Mux/1
  Mux/1 -> "lz{2,1}"/1

== matlab function Combined_net_5Class/If Action
Subsystem1/SOH estimation system/Subsystem1/MATLAB Function ==
function dV  = V_features(V_03,dv_mu_CC,dv_sig_CC)
dV = ((V_03(120-11)-V_03(1+10))-dv_mu_CC)/dv_sig_CC;
% if dV<-5 || dV>1
%     dV = 0;
% end
end

== matlab function Combined_net_5Class/If Action
Subsystem1/SOH estimation system/Subsystem1/MATLAB Function1 ==
function SOE  = SOE(I_03,V_03,SOE_mu_CC,SOE_sig_CC)

persistent  E1 E2 E3 E4 dE flag1 flag2 count SOE_reg
if isempty(E1)
    E1 = 0;
    E2 = 0;
    E3 = 0;
    E4 = 0;
    dE = 0;
    flag1 = 0;
    flag2 = 1;
    count = 0;
    SOE_reg = 0;
end

if I_03 ~= 0
    count = count+1;
end

if I_03(1)~=0 && flag1 ==0 && flag2 == 1
    E1 = I_03(1)*V_03(1);
    E2 = I_03(120)*V_03(120);
    flag1 = 1;
    flag2 = 0;
elseif I_03(1)~=0 && flag1 == 1 && flag2 == 0
    E3 = I_03(1)*V_03(1);
    E4 = I_03(120)*V_03(120);
    flag1 = 0;
    flag2 = 1;
end

SOE1 = zeros(1,120);

if count == 1
    SOE1(1) = 0;
elseif mod(count,2) == 1
    dE = (E1-E4)/2;
    SOE1(1) = SOE_reg+dE;
else
    dE = (E3-E2)/2;
    SOE1(1) = SOE_reg+dE;
end

time = linspace(1,120,120);
E = I_03.*V_03;
SOE_cum = cumtrapz(time,E);
k = 2;

for i = 1:119
    SOE1(k) = SOE_cum(i+1)-SOE_cum(i);
    k = k+1;
end

SOE_reg = SOE1(120);

SOE = (SOE1(120-11)-SOE_mu_CC)/SOE_sig_CC;
end

== matlab function Combined_net_5Class/If Action
Subsystem1/SOH estimation system/Subsystem1/MATLAB Function2 ==
function [SOC,dSOC] = SOC_features(SOC_03,SOC_mu_CC,SOC_sig_CC,dSOC_mu_CC,dSOC_sig_CC)
SOC = (SOC_03(120-11)-SOC_mu_CC)/SOC_sig_CC;
dSOC = ((SOC_03(120-11)-SOC_03(1+10))-dSOC_mu_CC)/dSOC_sig_CC;
if dSOC<-10
    dSOC = 0;
end
end

== matlab function Combined_net_5Class/If Action
Subsystem1/SOH estimation system/Subsystem1/MOVMEAN ==
function V_filt = filt(V)

V_filt = movmean(V,10);


end

== matlab function Combined_net_5Class/If Action
Subsystem1/SOH estimation system/Subsystem1/MOVMEAN1 ==
function I_filt = filt(I)

I_filt = movmean(I,10);


end
